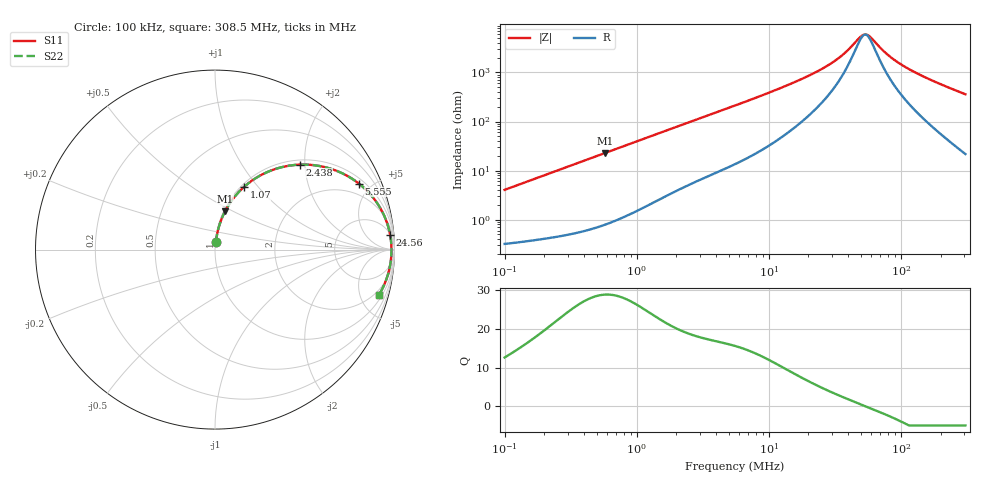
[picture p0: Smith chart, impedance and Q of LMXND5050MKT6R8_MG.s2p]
! LMXND5050MKT6R8_MG  S-PARAMETER MODEL  ( General Type )
! Model Generated by TAIYO YUDEN Corporation (https://www.yuden.co.jp/en/)
! Version 1.0
! TAIYO YUDEN Control No. 191023NI43SB-FBB
! Copyright(c) 2019 TAIYO YUDEN CO.,LTD. All Rights Reserved.
! Product Description (link to TY-COMPAS)
! https://ds.yuden.co.jp/TYCOMPAS/or/detail?pn=LMXND5050MKT6R8MMG&u=M
! Products Name : Inductors
! Characteristics :
!  Inductance : 6.8 uH , SRF(min) : 36 MHz , DC Resistance(max) : 0.312 Ohm
!  Rated Current : Saturation :1700 mA , Temp Rise : 1100 mA (40 degC)
!  Case Size : 4.9 x 4.9 / 0.193 x 0.193 [mm/inch] , Thickness : 1.2 / 0.047 [mm/inch]
!  (Conditions: Temperature = 25 degC , DC Bias Current/Voltage = 0A / 0V)
! External Node Assignments :
!  1  o---GGG---o  2
! GND o---------o GND
! Frequency Range : 0.1MHz  -  308.54851MHz  [ 402 STEP ]
# MHz S RI R 50
! Freq[MHz].  S11 Real  S11 Imag  S21 Real  S21 Imag  S12 Real  S12 Imag  S22 Real  S22 Imag
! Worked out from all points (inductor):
!   401 points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, 100 kHz to 308.5 MHz, reference 50 ohm
!   read as one part in series: L = 6.41 uH near 104.1 kHz
!   highest Q = 28.9 at 574 kHz (marker M1), where L = 6.31 uH
!   self-resonance near 53.81 MHz
!   S11 on the Smith chart (normalised r, x): 100 kHz: 1.01, +0.08; 1.07 MHz: 1.03, +0.84; 2.438 MHz: 1.10, +1.88; 5.555 MHz: 1.27, +4.21; 24.56 MHz: 5, +22; 308.5 MHz: 1.43, -7.16
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0.1  0.00481 0.0401  0.9952 -0.0401  0.9952 -0.0401  0.00481 0.0401
0.206082  0.0108 0.0812  0.9892 -0.0812  0.9892 -0.0812  0.0108 0.0812
0.384115  0.0281 0.1476  0.9719 -0.1476  0.9719 -0.1476  0.0281 0.1476
0.574021  0.0559 0.2131  0.9441 -0.2131  0.9441 -0.2131  0.0559 0.2131
1.069918  0.1602 0.3478  0.8398 -0.3478  0.8398 -0.3478  0.1602 0.3478
1.475446  0.2593 0.4167  0.7407 -0.4167  0.7407 -0.4167  0.2593 0.4167
2.437845  0.4714 0.4734  0.5286 -0.4734  0.5286 -0.4734  0.4714 0.4734
3.570664  0.6427 0.451  0.3573 -0.451  0.3573 -0.451  0.6427 0.451
5.554714  0.8016 0.368  0.1984 -0.368  0.1984 -0.368  0.8016 0.368
5.667415  0.8074 0.3634  0.1926 -0.3634  0.1926 -0.3634  0.8074 0.3634
9.945753  0.9192 0.2341  0.0808 -0.2341  0.0808 -0.2341  0.9192 0.2341
21.33651  0.9719 0.1014  0.0281 -0.1014  0.0281 -0.1014  0.9719 0.1014
24.55764  0.9757 0.0832  0.0243 -0.0832  0.0243 -0.0832  0.9757 0.0832
34.55277  0.9812 0.0442  0.0188 -0.0442  0.0188 -0.0442  0.9812 0.0442
39.76912  0.9824 0.0297  0.0176 -0.0297  0.0176 -0.0297  0.9824 0.0297
48.61598  0.9833 0.00984  0.0167 -0.00984  0.0167 -0.00984  0.9833 0.00984
52.68322  0.9834 0.00205  0.0166 -0.00205  0.0166 -0.00205  0.9834 0.00205
58.24905  0.9834 -0.00767  0.0166 0.00767  0.0166 0.00767  0.9834 -0.00767
81.95682  0.9817 -0.0419  0.0183 0.0419  0.0183 0.0419  0.9817 -0.0419
102.2213  0.9791 -0.0662  0.0209 0.0662  0.0209 0.0662  0.9791 -0.0662
138.1628  0.9724 -0.1042  0.0276 0.1042  0.0276 0.1042  0.9724 -0.1042
308.5485  0.9149 -0.2503  0.0851 0.2503  0.0851 0.2503  0.9149 -0.2503
